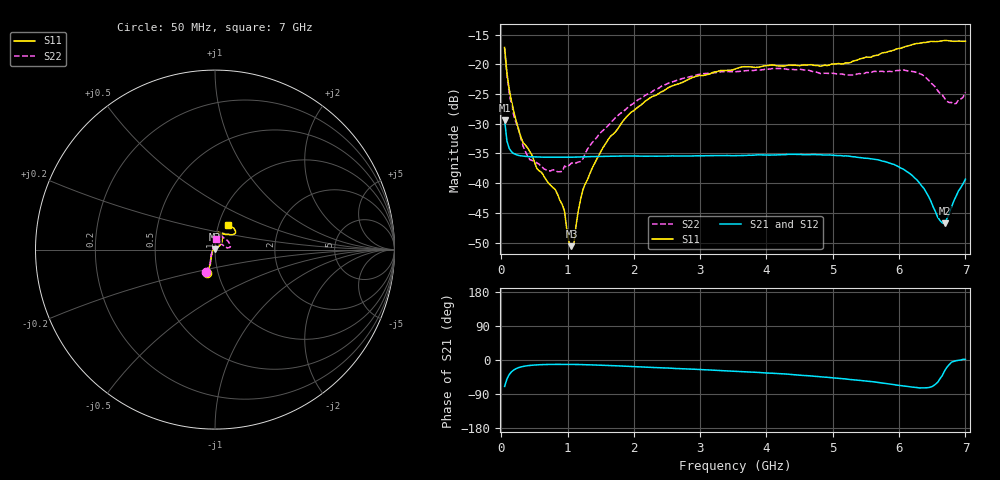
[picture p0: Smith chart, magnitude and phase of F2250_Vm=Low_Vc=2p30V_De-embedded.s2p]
! Integrated Device Technology
! Corporate Headquarters
! 6024 Silver Creek Valley Road
! San Jose, CA 95138  USA
! Phone:  1-408-284-8200
! Toll Free:  1-800-223-1366
! Webpage:  http://www.idt.com/
! Timing and RF Division
! 515 Groton Road, Suite 102
! Westford, MA 01886-6024
! Device:  F2250
! Description: Voltage Variable RF Attenuator
! Frequency:  50.0 -  6000.00 MHz
! Package:  3x3 mm Thin QFN Plastic Package: 16 pin
! Ports:  2 RF, 3 DC
!  Pin  1  = GND
!  Pin  2  = NC
!  Pin  3  = RF1  = Port 1
!  Pin  4  = NC
!  Pin  5  = GND
!  Pin  6  = GND
!  Pin  7  = GND
!  Pin  8  = GND
!  Pin  9  = NC
!  Pin 10  = RF2  = Port 2
!  Pin 11  = NC
!  Pin 12  = GND
!  Pin 13  = GND
!  Pin 14  = VCNTRL
!  Pin 15  = VDD
!  Pin 16  = VMODE
! Vcntrl:  2.300 Volts
! Vmode:  +0.000 Volts
! Vdd:  +3.30  Volts
! Current:  1.179 mA
! Data:  The device was measured on a the F2250 evaluation board which has
!  individual transmission lines to the RF pins.  Data was collected
!  using a calibrated network analyzer.  The evaluation board was
!  de-embedded using a TRL calibration technique.
!  The reference plane is the edge of the package pin.
! Misc:  SN 10
!  Action Tracker AT0258
! Date Measured:  2014-11-26
! Date:  2015-10-15  MJV
! Note:
!  Integrated Device Technology supplies this data as a sample of measured
!  data at the package pin for this product.  Your particular data for this
!  product may vary.
!  Data was taken at 25 degrees C.
!  Integrated Device Technology reserves the right to change this data at anytime.
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# GHz S dB R 50
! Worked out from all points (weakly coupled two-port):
!   201 points, 50 MHz to 7 GHz, reference 50 ohm
!   highest |S21| = -29.40 dB at 50 MHz (marker M1); lowest = -46.8 dB at 6.687 GHz (marker M2)
!   lowest |S11| = -50.6 dB at 1.058 GHz (marker M3), VSWR 1.01, Z = 49.8 + j0.248 ohm
!   |S11| at or under -10 dB: start of sweep to end of sweep
!   |S22| runs from -38.1 to -17.3 dB; largest |S21 - S12| = 6.1e-05
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0.05  -17.18 -108.6  -29.40 -69.7  -29.40 -69.7  -17.32 -110.8
0.08475  -21.44 -107.4  -32.90 -50.2  -32.89 -50.2  -21.81 -109.7
0.15425  -26.23 -116.6  -34.73 -31.0  -34.73 -31.1  -26.94 -121.5
0.29325  -32.20 -127.7  -35.40 -18.4  -35.40 -18.4  -32.36 -136.1
0.3975  -34.08 -141.7  -35.53 -15.0  -35.53 -15.0  -35.49 -159.3
0.91875  -43.57 158.3  -35.65 -11.5  -35.65 -11.5  -38.04 131.0
0.9535  -44.70 169.6  -35.65 -11.5  -35.65 -11.5  -37.13 129.0
1.023  -50.00 144.1  -35.64 -11.6  -35.64 -11.6  -37.00 113.1
1.05775  -50.60 122.6  -35.64 -11.6  -35.63 -11.6  -36.63 107.9
1.0925  -50.40 90.1  -35.63 -11.7  -35.63 -11.7  -36.59 103.1
1.162  -44.63 56.7  -35.60 -11.9  -35.61 -11.9  -36.45 92.2
1.2315  -41.09 44.3  -35.58 -12.1  -35.58 -12.1  -35.90 82.8
1.6485  -32.11 42.1  -35.49 -14.7  -35.49 -14.7  -29.88 62.9
1.96125  -28.05 42.2  -35.43 -17.2  -35.43 -17.3  -26.81 55.7
2.37825  -24.87 47.3  -35.45 -20.3  -35.44 -20.4  -24.01 56.0
3.525  -20.80 72.5  -35.38 -29.6  -35.38 -29.6  -21.26 74.4
4.7065  -20.17 72.4  -35.18 -42.6  -35.18 -42.6  -21.23 72.0
5.85325  -17.82 40.5  -36.61 -63.3  -36.61 -63.4  -21.18 22.5
6.27025  -16.51 40.1  -39.46 -72.6  -39.47 -72.7  -21.40 9.2
6.68725  -15.99 48.8  -46.77 -28.3  -46.76 -27.9  -25.73 28.0
6.861  -16.13 55.1  -42.16 -1.7  -42.13 -1.6  -26.58 57.9
7  -16.12 63.3  -39.34 1.5  -39.29 1.4  -24.71 83.3
